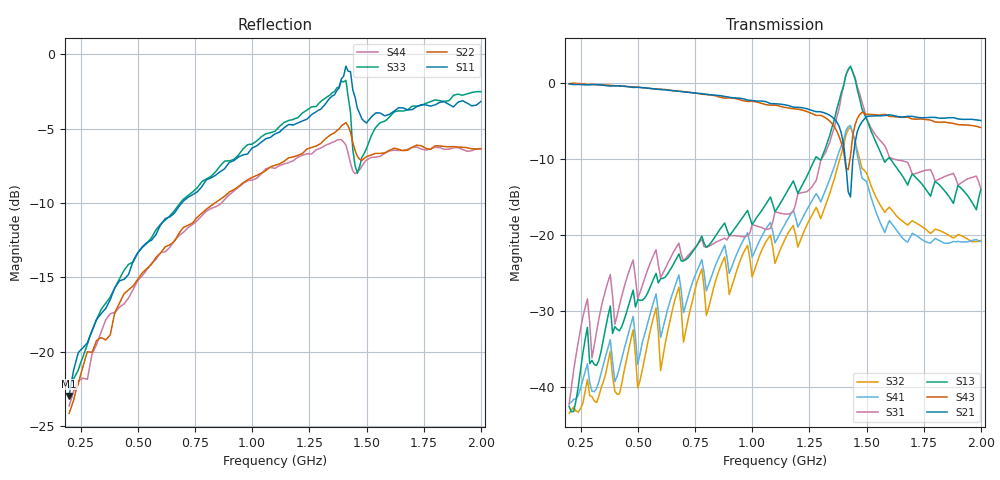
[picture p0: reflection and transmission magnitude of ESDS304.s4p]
! Created Mon Aug 27 11:03:46 2018
# hz S ma R 50
! 4 Port Network Data from SP1.SP block
! freq  magS11  angS11  magS12  angS12  magS13  angS13  magS14  angS14
!  magS21  angS21  magS22  angS22  magS23  angS23  magS24  angS24
!  magS31  angS31  magS32  angS32  magS33  angS33  magS34  angS34
!  magS41  angS41  magS42  angS42  magS43  angS43  magS44  angS44
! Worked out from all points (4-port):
!   181 points, 200 MHz to 2 GHz, reference 50 ohm
!   strongest paths, dB at 200 MHz, 650 MHz, 1.1 GHz, 1.55 GHz, 2 GHz:
!     S21: -0.1, -1.0, -2.7, -4.3, -4.9
!     S43: -0.1, -1.0, -2.9, -4.2, -5.9
!     S13: -42.6, -24.2, -17.0, -8.4, -14.0
!     S31: -42.4, -22.6, -17.0, -7.2, -14.0
!     S41: -42.2, -27.9, -21.1, -17.7, -20.9
!     S32: -43.5, -30.1, -23.8, -15.5, -20.7
!   lowest |S11| = -22.9 dB at 200 MHz (marker M1), VSWR 1.15, Z = 54 - j6.27 ohm
!   |S11| at or under -10 dB: start of sweep to 692.4 MHz
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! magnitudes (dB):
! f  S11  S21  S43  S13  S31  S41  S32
! 200 MHz  -22.9  -0.1  -0.1  -42.6  -42.4  -42.2  -43.5
! 380 MHz  -16.5  -0.4  -0.3  -29.4  -25.2  -33.8  -35.3
! 980 MHz  -6.7  -2.2  -2.4  -16.8  -20.1  -19.7  -21.4
! 1 GHz  -6.3  -2.3  -2.4  -18.7  -18.7  -23.0  -25.6
! 1.43 GHz  -1.2  -15.0  -9.6  2.2  2.2  -5.6  -5.8
! 1.48 GHz  -4.4  -5.1  -3.9  -3.4  -2.5  -12.5  -11.2
! 2 GHz  -3.2  -4.9  -5.9  -14.0  -14.0  -20.9  -20.7
